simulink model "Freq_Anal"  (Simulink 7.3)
settings: Solver=ode45  StartTime=0.0  StopTime=2000  RelTol=1e-3
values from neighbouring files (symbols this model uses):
  Api = [    [pitch_115.m]    (also in pitch_195.m; pitch_290.m; pitch_395.m; pitch_455.m)
  Bpi = [    [pitch_115.m]    (also in pitch_195.m; pitch_290.m; pitch_395.m; pitch_455.m)
  Cpi = [    [pitch_115.m]    (also in pitch_195.m; pitch_290.m; pitch_395.m; pitch_455.m)
  Dpi = [    [pitch_115.m]    (also in pitch_195.m; pitch_290.m; pitch_395.m; pitch_455.m)
undefined symbols (not defined in the file or in its folder): Kq

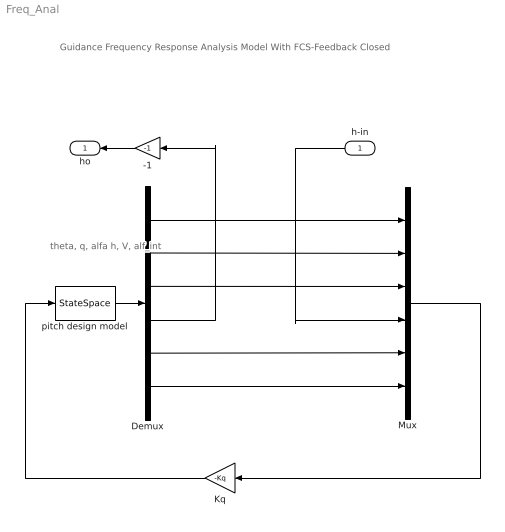
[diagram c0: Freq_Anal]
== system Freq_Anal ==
  note: Guidance Frequency Response Analysis Model With FCS-Feedback Closed
  note: theta, q, alfa h, V, alf_int
  h-in : Inport  OutDataType=sfix(16)  OutScaling=2^0
  -1 : Gain  Gain=-1  ParameterDataType=fixdt(1, 16)  ParameterScaling=2^0  OutDataType=fixdt(1, 16)  OutScaling=2^0
  Demux : Demux  Outputs=6
  Kq : Gain  Gain=-Kq  Multiplication=Matrix(K*u)  ParameterDataType=fixdt(1, 16)  ParameterScaling=2^0  OutDataType=fixdt(1, 16)  OutScaling=2^0
  Mux : Mux  Inputs=6
  pitch design model : StateSpace  A=Api  B=Bpi  C=Cpi  D=Dpi
  ho : Outport  OutDataType=sfix(16)  OutScaling=2^0
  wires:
  Kq/1 -> pitch design model/1
  -1/1 -> ho/1
  Demux/4 -> -1/1
  h-in/1 -> Mux/4
  pitch design model/1 -> Demux/1
  Demux/6 -> Mux/6
  Demux/5 -> Mux/5
  Demux/3 -> Mux/3
  Demux/2 -> Mux/2
  Demux/1 -> Mux/1
  Mux/1 -> Kq/1
